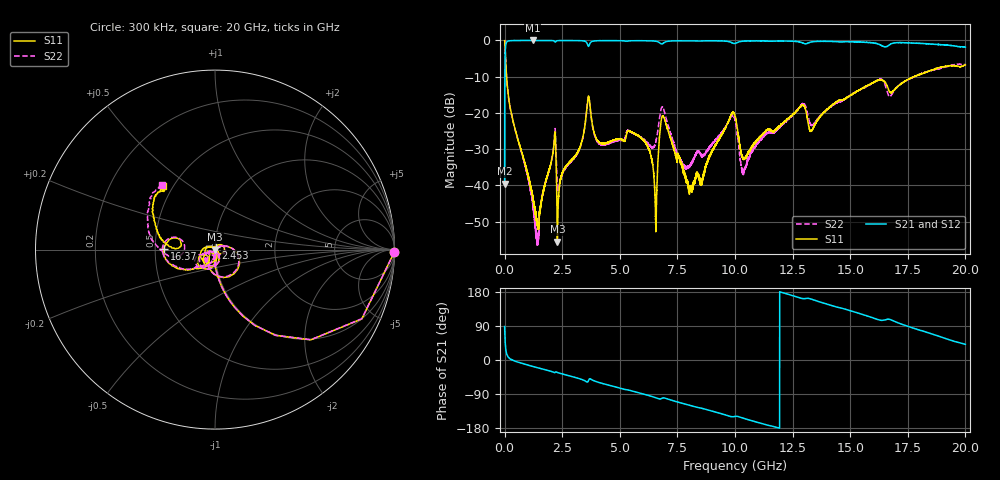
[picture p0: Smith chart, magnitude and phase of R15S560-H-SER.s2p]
!{R15S560}
!Johanson Technology Inc.
!www.johansontechnology.com
!Test Board Conditions:
!Substrate Type  RO4350B
!Substrate Thickness  20 mil
!Substrate Dk  3.66
!TL Type: GCPW
!TL Trace Width  34 mil
!TL Gap  10 mil
!Electrode orientation  Horizontal
!DUT TOPOLOGY	SERIES
!Mounting Pad LxW  26x52 mil
! Created Sat Feb  6 14:32:40 2021
# hz S ma R 50
! 2 Port Network Data from SP1.SP block
! freq  magS11  angS11  magS21  angS21  magS12  angS12  magS22  angS22
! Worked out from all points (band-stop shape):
!   20001 points, 300 kHz to 20 GHz, reference 50 ohm
!   highest |S21| = 0.00 dB at 1.218 GHz (marker M1); lowest = -39.5 dB at 300 kHz (marker M2)
!   |S21| within 3 dB of the highest: 28.54 MHz to end of sweep
!   lowest |S11| = -55.6 dB at 2.291 GHz (marker M3), VSWR 1.00, Z = 50.2 + j0.0276 ohm
!   |S11| at or under -10 dB: 84.9 MHz to 17.78 GHz (17.69 GHz wide, 198 % of centre)
!   |S22| runs from -56.8 to 0.0 dB; largest |S21 - S12| = 0.015
!   S11 on the Smith chart (normalised r, x): 300 kHz: open; 2.453 GHz: 1.01, +0.02; 16.37 GHz: 0.56, +0.01; 20 GHz: 0.44, +0.40
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300000  0.9983 -0.9  0.01056 88.3  0.0106 89.2  0.9991 -0.8
1.253e8  0.2204 -79.0  0.9747 10.8  0.9744 10.8  0.2212 -79.0
1.2183e9  0.006904 -121.7  0.9998 -17.0  0.9982 -17.0  0.005878 -98.8
1.4193e9  0.002958 -163.9  0.9987 -20.2  0.9986 -20.2  0.001913 -25.3
2.1333e9  0.03443 53.0  0.9888 -32.5  0.9899 -32.4  0.03571 35.6
2.2913e9  0.001663 9.5  0.9922 -32.8  0.9929 -32.8  0.00972 -33.4
2.4533e9  0.01321 64.6  0.9961 -35.9  0.9963 -35.9  0.01311 28.6
3.3343e9  0.0388 29.2  0.9914 -51.1  0.9909 -51.0  0.038 30.0
3.6483e9  0.1711 -58.9  0.8296 -52.9  0.8298 -52.9  0.1661 -59.9
4.1913e9  0.03815 -140.1  0.9932 -60.9  0.9936 -61.0  0.03684 -152.4
5.9523e9  0.04393 163.3  0.9924 -88.6  0.9924 -88.7  0.04503 -153.6
6.5403e9  0.005682 105.8  0.978 -99.2  0.9782 -99.1  0.03706 -101.6
6.6673e9  0.02541 -60.4  0.9553 -102.0  0.9551 -101.9  0.06211 -86.4
6.9013e9  0.08836 -154.6  0.9237 -99.9  0.9227 -99.9  0.1128 -138.9
8.0833e9  0.008943 46.5  0.9903 -120.4  0.9897 -120.4  0.01891 -95.3
1.00003e10  0.09226 -134.7  0.9102 -148.9  0.9099 -148.8  0.08084 -134.3
1.03763e10  0.02305 -120.9  0.9781 -153.9  0.979 -153.9  0.01478 -110.3
1.28913e10  0.1258 -123.2  0.9356 162.6  0.9373 162.8  0.1314 -131.6
1.33343e10  0.05749 -129.1  0.9564 160.3  0.9565 160.1  0.06723 -143.1
1.63663e10  0.2841 179.1  0.8474 104.6  0.8447 104.7  0.2912 175.8
1.66673e10  0.2072 163.8  0.855 107.5  0.844 107.7  0.1739 170.2
2e10  0.4593 129.3  0.8086 41.1  0.8002 40.8  0.4643 129.3
